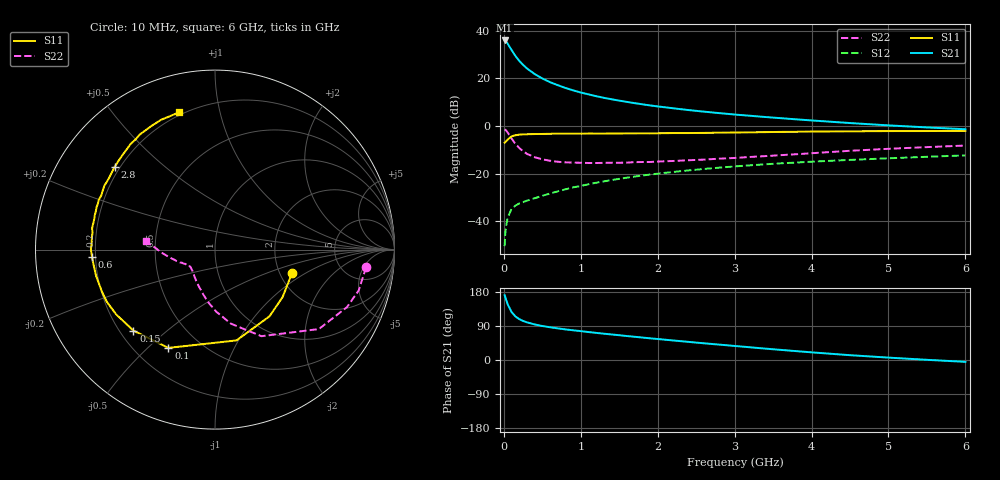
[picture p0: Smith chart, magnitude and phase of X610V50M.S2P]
! SIEMENS Small Signal Semiconductors
! BFP193W
! Si NPN RF Bipolar Junction Transistor in SOT343
! VCE = 10 V  IC = 50 mA
! Common Emitter S-Parameters:  April 1994
# GHz  S  MA  R  50
!  f  S11  S21  S12  S22
! GHz  MAG  ANG  MAG  ANG  MAG  ANG  MAG  ANG
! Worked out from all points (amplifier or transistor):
!   40 points, 10 MHz to 6 GHz, reference 50 ohm
!   highest |S21| = 35.9 dB at 10 MHz (marker M1)
!   |S21| within 3 dB of that: start of sweep to 80.95 MHz
!   unconditionally stable (mu >= 1): 743.2 MHz to 4.983 GHz
!   at 200 MHz: K = 0.52, MSG = 29.9 dB, |S12| = -32.5 dB
!   at 1.5 GHz: K = 1.11, MAG = 14.4 dB, |S12| = -22.2 dB
!   at 6 GHz: K = 0.97, MSG = 5.5 dB, |S12| = -12.3 dB
!   S11 on the Smith chart (normalised r, x): 10 MHz: 2.32, -0.77; 100 MHz: 0.34, -0.58; 150 MHz: 0.25, -0.39; 600 MHz: 0.19, -0.03; 2.8 GHz: 0.18, +0.35; 6 GHz: 0.18, +0.76
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0.01  0.4486 -17.1  62.65 171.1  0.003 66.4  0.8473 -6.7
0.02  0.4604 -35.2  61.34 165.1  0.0059 67.5  0.8323 -15.9
0.03  0.48 -50.8  59.32 158.7  0.008 67.0  0.8023 -23.5
0.05  0.52 -76.7  53.54 146.8  0.0119 60.4  0.7287 -37.4
0.1  0.6062 -115.4  39.5 126.9  0.0182 48.6  0.5475 -61.8
0.15  0.6404 -135.2  29.74 115.0  0.0213 44.1  0.4225 -77.8
0.2  0.6583 -146.7  23.38 108.0  0.0237 43.5  0.3455 -88.9
0.25  0.6693 -154.2  19.25 103.0  0.0252 43.1  0.2971 -97.1
0.3  0.6721 -159.6  16.2 99.4  0.0271 44.7  0.2605 -104.2
0.4  0.6784 -167.4  12.37 93.9  0.0304 47.7  0.2217 -114.4
0.5  0.6817 -172.8  9.983 89.7  0.0343 51.2  0.2001 -122.3
0.6  0.6866 -176.7  8.342 86.4  0.0382 53.0  0.1866 -128.3
0.8  0.6883 177.1  6.303 80.8  0.0468 56.3  0.1729 -136.1
1.1  0.6952 170.1  4.626 73.8  0.0599 58.7  0.1674 -143.5
1.3  0.6938 166.0  3.915 69.4  0.0689 59.1  0.1686 -146.1
1.6  0.7008 160.3  3.212 63.2  0.0823 58.8  0.1706 -149.1
2.2  0.7118 150.0  2.36 51.6  0.1086 56.1  0.1846 -154.7
2.8  0.7248 140.3  1.867 40.6  0.1337 52.3  0.2064 -159.4
3.2  0.7374 134.2  1.643 33.6  0.1494 49.4  0.2241 -163.6
4.5  0.7743 117.3  1.155 12.7  0.1943 40.0  0.3022 -177.2
5.5  0.7844 108.8  0.935 0.5  0.226 33.6  0.3607 175.5
6  0.791 104.6  0.856 -4.9  0.2421 30.9  0.3892 173.0
